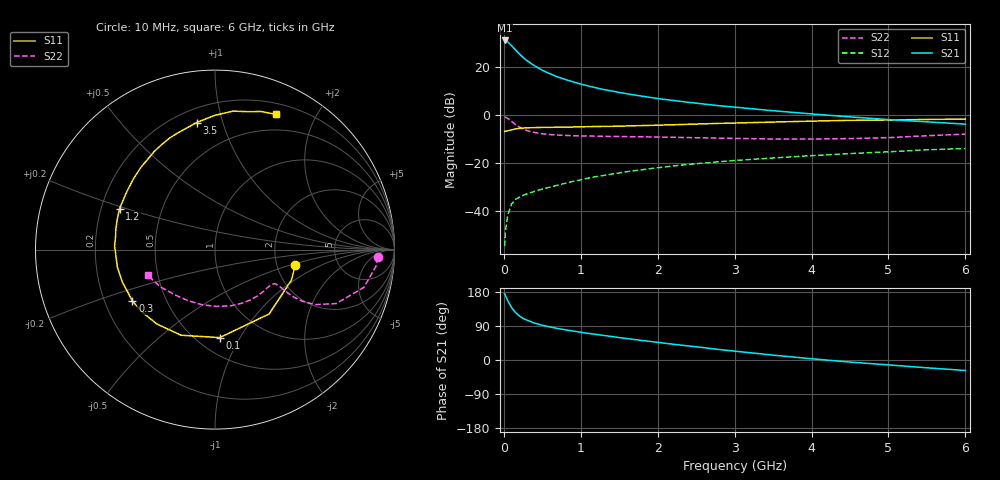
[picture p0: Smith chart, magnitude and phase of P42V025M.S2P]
! SIEMENS Small Signal Semiconductors
! BFP182
! Si NPN RF Bipolar Junction Transistor in SOT143
! VCE = 2 V  IC = 25 mA
! Common Emitter S-Parameters:  March  1996
# GHz  S  MA  R  50
!  f  S11  S21  S12  S22
! GHz  MAG  ANG  MAG  ANG  MAG  ANG  MAG  ANG
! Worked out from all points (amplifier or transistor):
!   36 points, 10 MHz to 6 GHz, reference 50 ohm
!   highest |S21| = 31.3 dB at 10 MHz (marker M1)
!   |S21| within 3 dB of that: start of sweep to 123.2 MHz
!   unconditionally stable (mu >= 1): start of sweep to 11.5 MHz; 428 MHz to end of sweep
!   at 250 MHz: K = 0.72, MSG = 28.9 dB, |S12| = -33.6 dB
!   at 1.4 GHz: K = 1.43, MAG = 13.5 dB, |S12| = -24.7 dB
!   at 6 GHz: K = 1.05, MAG = 3.7 dB, |S12| = -14.0 dB
!   S11 on the Smith chart (normalised r, x): 10 MHz: 2.54, -0.54; 100 MHz: 0.64, -0.83; 300 MHz: 0.32, -0.26; 1.2 GHz: 0.28, +0.19; 3.5 GHz: 0.28, +0.83; 6 GHz: 0.32, +1.50
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0.01  0.4555 -10.7  36.59 175.1  0.0018 75.7  0.9073 -2.7
0.02  0.4586 -21.6  36.53 170.6  0.0036 76.8  0.9019 -5.9
0.05  0.4685 -49.9  34.4 156.6  0.0079 75.0  0.8563 -14.2
0.1  0.491 -86.9  28.41 138.5  0.0137 58.0  0.7391 -24.0
0.15  0.5132 -111.6  23.3 125.7  0.0171 52.5  0.6368 -28.8
0.2  0.5261 -128.0  19.26 116.6  0.019 49.0  0.5633 -30.6
0.25  0.5351 -139.5  16.11 109.9  0.0209 48.4  0.5111 -31.1
0.3  0.5419 -148.1  13.85 105.1  0.0224 48.6  0.4743 -30.8
0.4  0.5467 -160.6  10.77 97.4  0.0253 49.7  0.431 -30.0
0.5  0.5529 -169.5  8.693 91.8  0.0283 50.3  0.4062 -29.6
0.6  0.5533 -176.4  7.343 87.2  0.031 52.1  0.3914 -29.5
0.7  0.5597 177.8  6.293 83.2  0.0341 53.5  0.3816 -29.9
0.8  0.5583 173.1  5.57 79.6  0.0374 54.5  0.3753 -30.7
1.1  0.573 160.5  4.071 70.2  0.0482 56.2  0.3647 -34.0
1.2  0.5783 156.7  3.724 67.5  0.0514 56.1  0.362 -35.5
1.7  0.5985 140.4  2.633 54.0  0.0686 54.8  0.3526 -44.1
2.2  0.6267 127.0  2.031 41.6  0.086 51.8  0.3436 -54.4
2.8  0.6712 112.2  1.573 27.6  0.1056 46.7  0.3287 -68.7
3.5  0.7154 98.2  1.234 12.9  0.1266 40.5  0.3166 -88.2
4.5  0.7779 82.6  0.918 -5.5  0.1563 31.7  0.3221 -118.3
5.5  0.8112 71.5  0.723 -20.6  0.1879 22.7  0.3698 -146.2
6  0.8259 65.9  0.647 -27.7  0.2002 17.3  0.3995 -158.9
